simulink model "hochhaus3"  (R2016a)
settings: Solver=ode45  StartTime=0.0  StopTime=5  MaxStep=1e-2  RelTol=1e-3

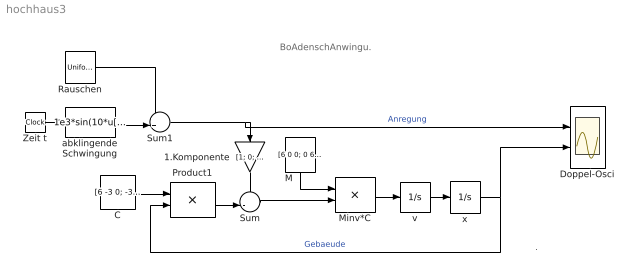
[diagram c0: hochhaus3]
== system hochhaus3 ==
  note: .
  note: BoAdenschAnwingu.
  1.Komponente : Gain  Gain=[1; 0; 0]
  C : Constant  Value=[6 -3 0; -3 4 -1; 0 -1 1]*1e6  VectorParams1D=off
  Doppel-Osci : Scope  NumInputPorts=2
  M : Constant  Value=[6 0 0; 0 6 0; 0 0 1]*1e3  VectorParams1D=off
  Minv*C : Product  Inputs=/*  Multiplication=Matrix(*)
  Product1 : Product  Multiplication=Matrix(*)
  Rauschen : UniformRandomNumber  Minimum=-100  Maximum=100  SampleTime=0
  Sum : Sum  Inputs=+-|
  Sum1 : Sum  Inputs=++|
  Zeit t : Clock
  abklingende Schwingung : Fcn  Expr=1e3*sin(10*u[1])*exp(-1.1*u[1])
  v : Integrator  InitialCondition=[0; 0; 0]
  x : Integrator  InitialCondition=[0; 0; 0]
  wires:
  v/1 -> x/1
  x/1 -> Product1/2, Doppel-Osci/2  "Gebaeude"
  Product1/1 -> Sum/2
  Zeit t/1 -> abklingende Schwingung/1
  abklingende Schwingung/1 -> Sum1/2
  Rauschen/1 -> Sum1/1
  Sum1/1 -> 1.Komponente/1, Doppel-Osci/1  "Anregung"
  1.Komponente/1 -> Sum/1
  C/1 -> Product1/1
  Minv*C/1 -> v/1
  Sum/1 -> Minv*C/2
  M/1 -> Minv*C/1
